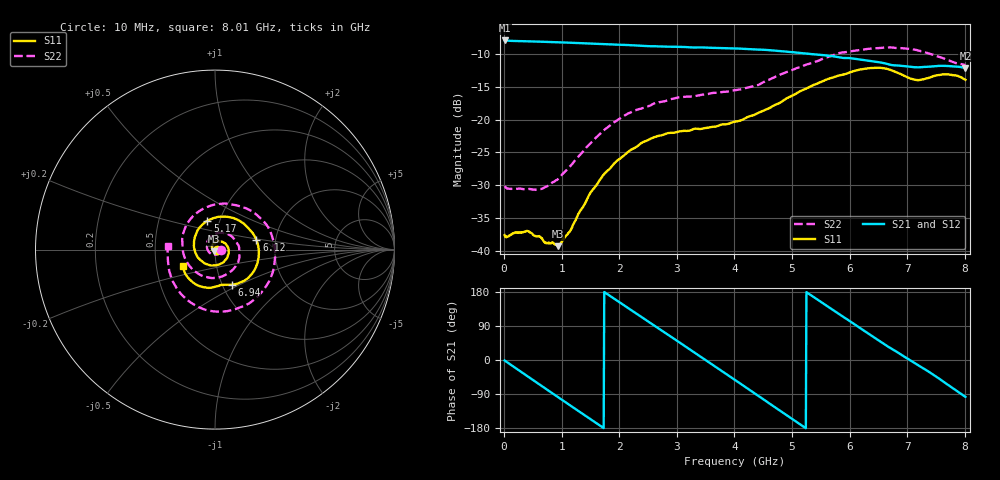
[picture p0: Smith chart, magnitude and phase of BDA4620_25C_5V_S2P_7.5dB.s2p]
!Agilent Technologies,E5071B,MY42404982,A.09.10
!Date: Wed May 06 08:59:42 2026
!Data & Calibration Information:
!Freq	S11:SOLT2(ON)	S21:SOLT2(ON)	S12:SOLT2(ON)	S22:SOLT2(ON)
# Hz S RI R 50
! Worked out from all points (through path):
!   801 points, 10 MHz to 8.01 GHz, reference 50 ohm
!   highest |S21| = -7.94 dB at 10 MHz (marker M1); lowest = -12.1 dB at 8.01 GHz (marker M2)
!   group delay of S21, straight-line fit = 283 ps
!   lowest |S11| = -39.3 dB at 930 MHz (marker M3), VSWR 1.02, Z = 49.4 - j0.887 ohm
!   |S11| at or under -10 dB: start of sweep to end of sweep
!   |S22| runs from -30.7 to -9.0 dB; largest |S21 - S12| = 0.0021
!   S11 on the Smith chart (normalised r, x): 10 MHz: 1.03, -0.00; 5.17 GHz: 0.87, +0.29; 6.12 GHz: 1.59, +0.18; 6.94 GHz: 1.11, -0.45; 8.01 GHz: 0.69, -0.13
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1e7  0.0131 -0.000762  0.4008 -0.00868  0.4011 -0.00876  0.031 -0.00237
5.2e8  0.00934 -0.00914  0.228 -0.3208  0.2279 -0.3214  0.00727 -0.0284
9.3e8  -0.00606 -0.00898  -0.0485 -0.3854  -0.0487 -0.3858  -0.0301 -0.0178
1.35e9  -0.0173 0.0119  -0.2954 -0.2424  -0.2957 -0.2425  -0.045 0.0328
1.65e9  -0.00864 0.0328  -0.3729 -0.056  -0.3733 -0.0562  -0.0223 0.0732
1.94e9  0.0131 0.0457  -0.3475 0.1345  -0.348 0.1349  0.0252 0.0939
2.33e9  0.0509 0.0376  -0.1768 0.3208  -0.1771 0.3212  0.0977 0.069
2.68e9  0.075 0.00507  0.0409 0.3588  0.0413 0.3591  0.1351 0.00486
3e9  0.0714 -0.0365  0.2258 0.2788  0.2262 0.2786  0.1284 -0.0707
3.39e9  0.0361 -0.0766  0.3477 0.0692  0.3483 0.0686  0.0546 -0.1428
3.69e9  -0.00849 -0.0885  0.3313 -0.1177  0.331 -0.1185  -0.0352 -0.1559
4.01e9  -0.0617 -0.0739  0.211 -0.2767  0.2111 -0.2774  -0.1294 -0.1063
4.53e9  -0.1174 0.016  -0.0971 -0.3257  -0.0975 -0.3259  -0.1814 0.0729
4.87e9  -0.1011 0.099  -0.2605 -0.2035  -0.2608 -0.2035  -0.1078 0.1996
5.17e9  -0.0423 0.161  -0.3184 -0.0404  -0.3186 -0.04  0.0169 0.2528
5.35e9  0.0118 0.1811  -0.3092 0.0611  -0.3091 0.0615  0.1018 0.2501
5.75e9  0.1443 0.1557  -0.1846 0.239  -0.1845 0.2398  0.2706 0.1578
6.12e9  0.2312 0.0525  -0.0026 0.2894  -0.00183 0.29  0.3354 -0.0271
6.68e9  0.1773 -0.1642  0.2181 0.1475  0.2191 0.1474  0.2048 -0.2894
6.94e9  0.0922 -0.1957  0.252 0.0434  0.2527 0.0427  0.071 -0.3423
7.5e9  -0.0401 -0.213  0.1853 -0.1757  0.1852 -0.1768  -0.2039 -0.2287
8.01e9  -0.1776 -0.0941  -0.0315 -0.2458  -0.0321 -0.2468  -0.2595 0.0211
